(* Logix 5000 AddOnInstructionDefinition export; software revision 16.04 *)

TYPE AKD_Status :   // All connections to the drive ethernet module are established and data is successfully transferring.
STRUCT
   Profile_In_Progress : BOOL;   // Profile Move In Progress
   Block_In_Execution : BOOL;   // Block In Execution
   On_Target_Position : BOOL;   // On Target Position (1=Current Position Equals Last Target Position)
   General_Fault : BOOL;   // General Fault
   Current_Direction : BOOL;   // Current Motor Direction (0=Reverse, 1=Forward)
   Home_Level : BOOL;   // Level of Home Input
   Reg_Level : BOOL;   // Level of Registration Input
   Enable : BOOL;   // State of Enable Output
   Fault_Input_Fault : BOOL;   // Fault Input Active
   Fwd_Limit : BOOL;   // Forward Input Active
   Rev_Limit : BOOL;   // Reverse Input Active
   Positive_Limit : BOOL;   // Positive Software Limit Exceeded
   Negative_Limit : BOOL;   // Negative Software Limit Exceeded
   FE_Fault : BOOL;   // Following Error Fault
   Block_Fault : BOOL;   // Block Execution Fault
   Load_Complete : BOOL;   // Command Message Successfully Loaded
END_STRUCT
END_TYPE

TYPE AKD_Axis :   // Axis Data:
STRUCT
   Control : AKD_Control;   // Control bits to send to the drive
   Status : AKD_Status;   // Status bits received from the drive
   Input : AB:ETHERNET_MODULE_SINT_64Bytes:I:0;   // Data from the drive
   Output : AB:ETHERNET_MODULE_SINT_64Bytes:O:0;   // Data to the drive
   ResponseMsgType : SINT;   // Response type contained in latest IO response from drive. Used to check for errors
   CommandTimeout : INT;   // Time to allow for command response from drive. Dependent on scan rate and communicaiton rate
   PositionFeedback : DINT;   // Actual Position Value
   VelocityFeedback : DINT;   // Actual Velocity Value
END_STRUCT
END_TYPE

TYPE AKD_Control :   // Send Explicit Message
STRUCT
   Load_Data_Start_Profile : BOOL;   // Load Command Data / Start Profile Move
   Start_Block : BOOL;   // Execute Command block or block chain
   Incremental : BOOL;   // Incremental Position (0=Absolute, 1=Incremental)
   Direction : BOOL;   // Direction in Velocity Mode (0=Reverse, 1=Forward)
   Smooth_Stop : BOOL;   // Smooth / Controlled Stop w/ Deceleration
   Hard_Stop : BOOL;   // Hard / Immediate Stop
   Reg_Arm : BOOL;   // Arm the Registration Input
   Enable : BOOL;   // Enable Output
END_STRUCT
END_TYPE

ADD_ON_INSTRUCTION AKD_Set_Attribute   (* revision 2.1, ExecutePrescan, ExecuteEnableInFalse *)
// Set Position Controller Attribute
// Revision note:
// Don't error if Command_Timeout preset is 0
VAR_OUTPUT
   DN : BOOL; {visible}   // Command Successful
   ER : BOOL; {visible}   // Error
END_VAR
VAR_IN_OUT
   Axis : AKD_Axis; {required}
END_VAR
VAR_INPUT
   Attribute_Number : INT; {visible}   // Attribute Number (see help for options)
   Attribute_Value : DINT; {required}   // Attribute Value
END_VAR
VAR
   Command_Timeout : TIMER;   // Timeout Timer
   Command_Message_Type : SINT;   // Command Message Type
   Command_Axis_Number : SINT;   // Command Axis Number
   Step : SINT;
   Command_Bytes : SINT[8];
   OS_LoadStart : BOOL;
END_VAR

ROUTINE EnableInFalse   (* ladder *)
// EnableIn_False
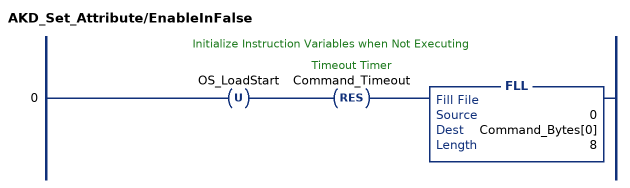
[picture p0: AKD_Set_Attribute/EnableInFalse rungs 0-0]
   // Initialize Instruction Variables when Not Executing
   0: OTU(OS_LoadStart)RES(Command_Timeout)FLL(0,Command_Bytes[0],8);
END_ROUTINE

ROUTINE Logic   (* ladder *)
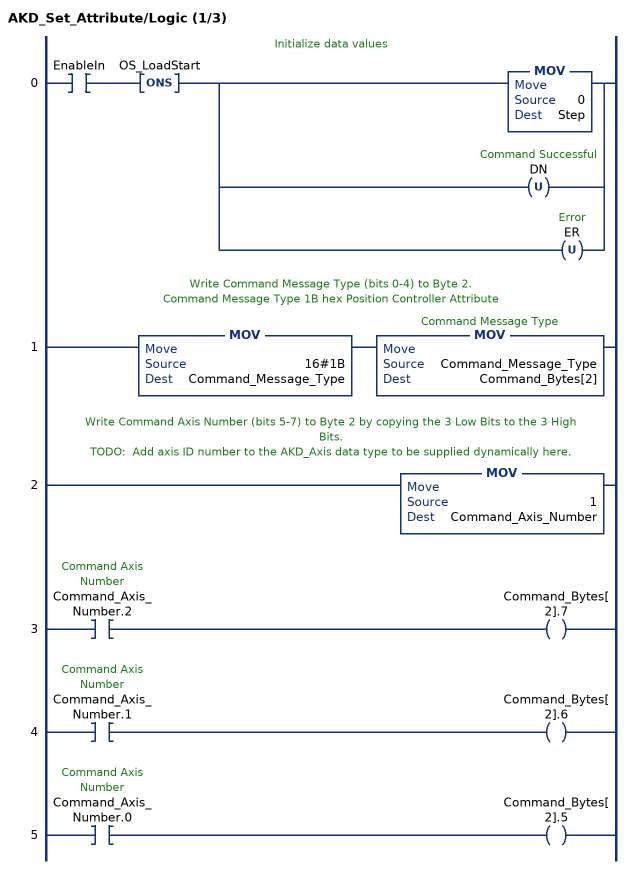
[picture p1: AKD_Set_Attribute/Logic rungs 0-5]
   // Initialize data values
   0: XIC(EnableIn)ONS(OS_LoadStart)[MOV(0,Step) ,OTU(DN) ,OTU(ER) ];
   // Write Command Message Type (bits 0-4) to Byte 2.
   // Command Message Type 1B hex Position Controller Attribute
   1: MOV(16#1B,Command_Message_Type)MOV(Command_Message_Type,Command_Bytes[2]);
   // Write Command Axis Number (bits 5-7) to Byte 2 by copying the 3 Low Bits to the 3 High Bits.
   // TODO:  Add axis ID number to the AKD_Axis data type to be supplied dynamically here.
   2: MOV(1,Command_Axis_Number);
   3: XIC(Command_Axis_Number.2)OTE(Command_Bytes[2].7);
   4: XIC(Command_Axis_Number.1)OTE(Command_Bytes[2].6);
   5: XIC(Command_Axis_Number.0)OTE(Command_Bytes[2].5);
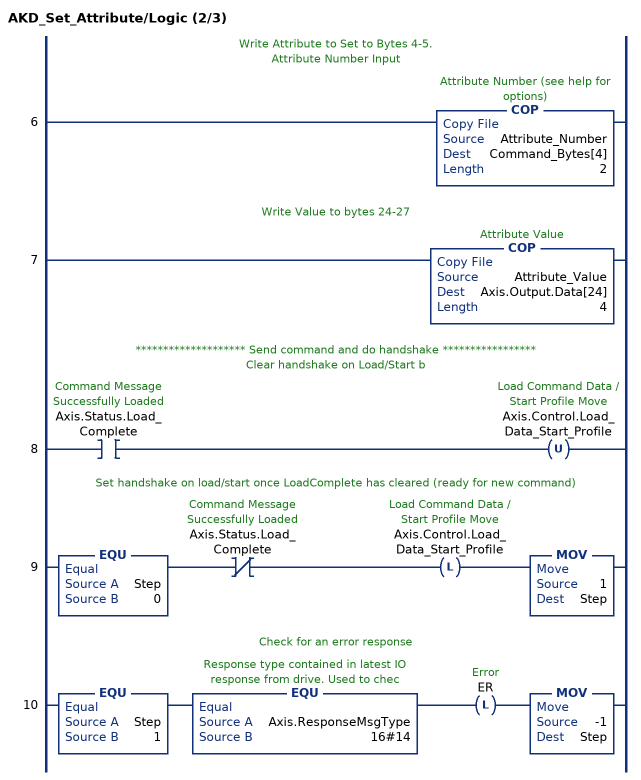
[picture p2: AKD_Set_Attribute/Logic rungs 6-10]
   // Write Attribute to Set to Bytes 4-5.
   // Attribute Number Input
   6: COP(Attribute_Number,Command_Bytes[4],2);
   // Write Value to bytes 24-27
   7: COP(Attribute_Value,Axis.Output.Data[24],4);
   // ******************** Send command and do handshake *****************
   // Clear handshake on Load/Start b
   8: XIC(Axis.Status.Load_Complete)OTU(Axis.Control.Load_Data_Start_Profile);
   // Set handshake on load/start once LoadComplete has cleared (ready for new command)
   9: EQU(Step,0)XIO(Axis.Status.Load_Complete)OTL(Axis.Control.Load_Data_Start_Profile)MOV(1,Step);
   // Check for an error response
   10: EQU(Step,1)EQU(Axis.ResponseMsgType,16#14)OTL(ER)MOV(-1,Step);
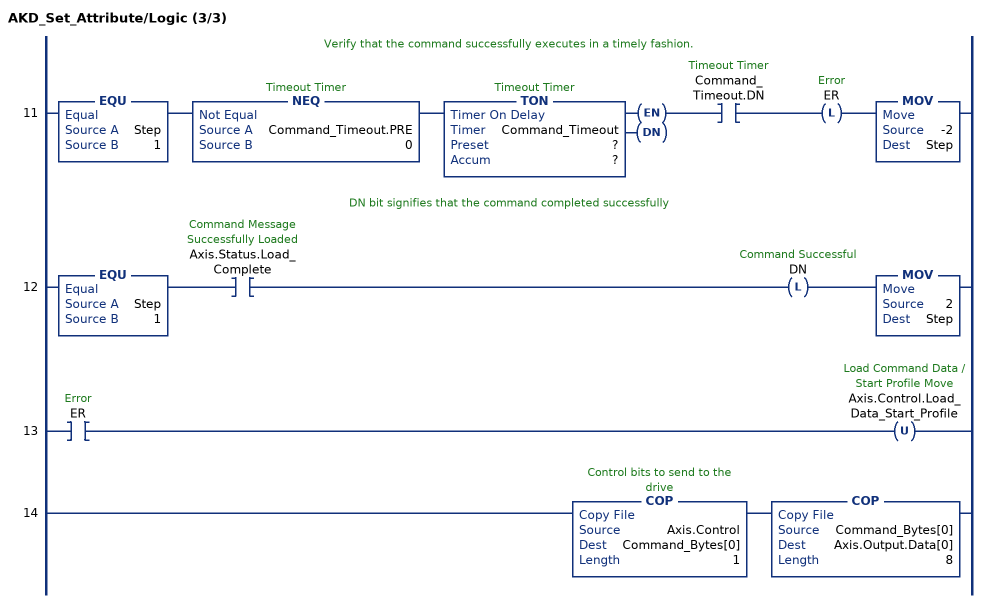
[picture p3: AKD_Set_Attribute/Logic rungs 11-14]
   // Verify that the command successfully executes in a timely fashion.
   11: EQU(Step,1)NEQ(Command_Timeout.PRE,0)TON(Command_Timeout,?,?)XIC(Command_Timeout.DN)OTL(ER)MOV(-2,Step);
   // DN bit signifies that the command completed successfully
   12: EQU(Step,1)XIC(Axis.Status.Load_Complete)OTL(DN)MOV(2,Step);
   13: XIC(ER)OTU(Axis.Control.Load_Data_Start_Profile);
   14: COP(Axis.Control,Command_Bytes[0],1)COP(Command_Bytes[0],Axis.Output.Data[0],8);
END_ROUTINE

ROUTINE Prescan   (* ladder *)
// Prescan
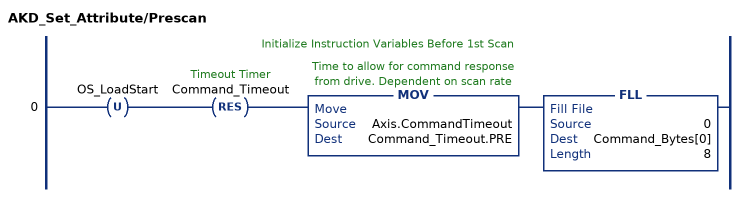
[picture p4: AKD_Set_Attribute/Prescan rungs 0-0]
   // Initialize Instruction Variables Before 1st Scan
   0: OTU(OS_LoadStart)RES(Command_Timeout)MOV(Axis.CommandTimeout,Command_Timeout.PRE)FLL(0,Command_Bytes[0],8);
END_ROUTINE
END_ADD_ON_INSTRUCTION

ADD_ON_INSTRUCTION AKD_Set_Units   (* revision 2.2, ExecutePrescan, ExecuteEnableInFalse *)
// Set Drive Units for Motion Commands
// Revision note:
// Clean up instruction, especially for error recovery.
VAR_IN_OUT
   Axis : AKD_Axis; {required}
END_VAR
VAR_INPUT
   Units : SINT; {required}   // Drive Units (0=Counts 16 bit)
END_VAR
VAR_OUTPUT
   DN : BOOL; {visible}   // Command Successfully Initiated
   ER : BOOL; {visible}   // Error
END_VAR
VAR
   Set_POSUNIT : AKD_Set_Attribute;
   Set_PROFUNIT : AKD_Set_Attribute;
   Step : SINT;   // Sequence Step Number
   OS_Start_Sequence : BOOL;
   Profile_Ratio : DINT;   // The number of actual feedback counts per second or second2 equal to one velocity or acceleration unit
   Position_Ratio : DINT;   // The number of actual position feedback counts equal to one position unit
   Invalid_Input : BOOL;   // Invalid Units Input
END_VAR

ROUTINE EnableInFalse   (* ladder *)
// EnableIn_False
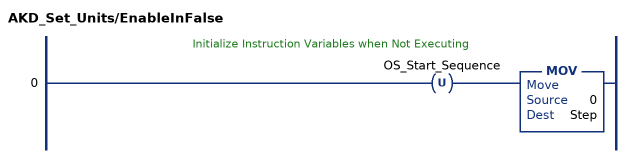
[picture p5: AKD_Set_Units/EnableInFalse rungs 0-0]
   // Initialize Instruction Variables when Not Executing
   0: OTU(OS_Start_Sequence)MOV(0,Step);
END_ROUTINE

ROUTINE Logic   (* ladder *)
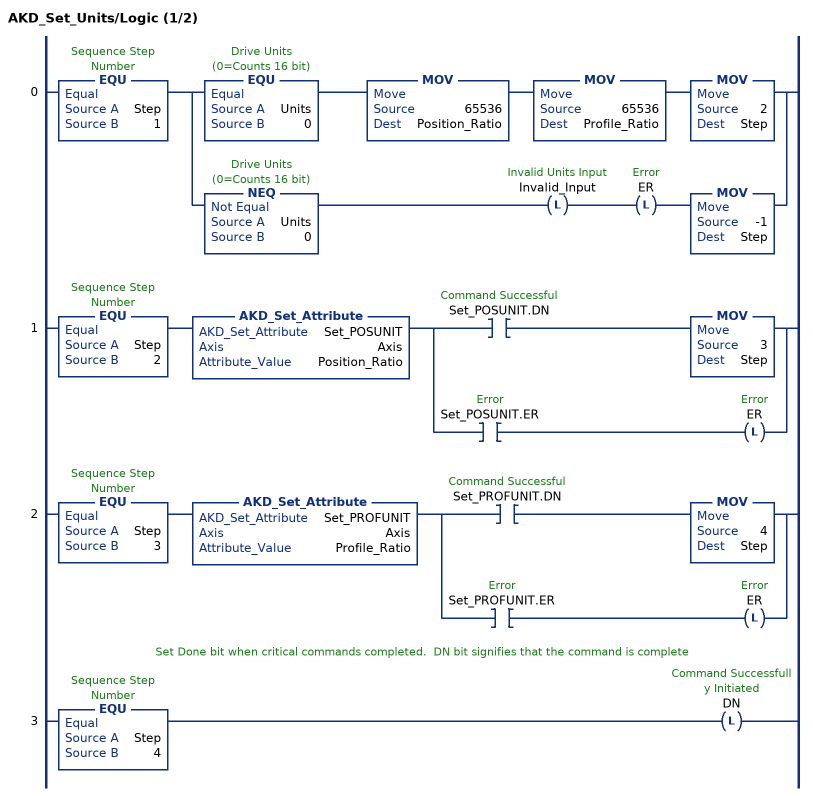
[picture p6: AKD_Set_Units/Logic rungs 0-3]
   0: EQU(Step,1)[EQU(Units,0) MOV(65536,Position_Ratio) MOV(65536,Profile_Ratio) MOV(2,Step) ,NEQ(Units,0) OTL(Invalid_Input) OTL(ER) MOV(-1,Step) ];
   1: EQU(Step,2)AKD_Set_Attribute(Set_POSUNIT,Axis,Position_Ratio)[XIC(Set_POSUNIT.DN) MOV(3,Step) ,XIC(Set_POSUNIT.ER) OTL(ER) ];
   2: EQU(Step,3)AKD_Set_Attribute(Set_PROFUNIT,Axis,Profile_Ratio)[XIC(Set_PROFUNIT.DN) MOV(4,Step) ,XIC(Set_PROFUNIT.ER) OTL(ER) ];
   // Set Done bit when critical commands completed.  DN bit signifies that the command is complete
   3: EQU(Step,4)OTL(DN);
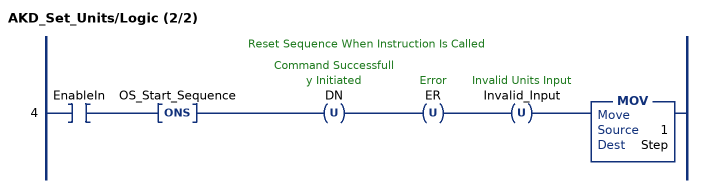
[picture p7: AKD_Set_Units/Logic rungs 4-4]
   // Reset Sequence When Instruction Is Called
   4: XIC(EnableIn)ONS(OS_Start_Sequence)OTU(DN)OTU(ER)OTU(Invalid_Input)MOV(1,Step);
END_ROUTINE

ROUTINE Prescan   (* ladder *)
// Prescan
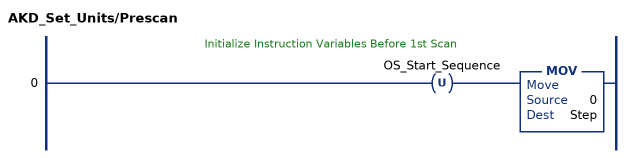
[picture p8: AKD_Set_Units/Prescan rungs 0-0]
   // Initialize Instruction Variables Before 1st Scan
   0: OTU(OS_Start_Sequence)MOV(0,Step);
END_ROUTINE
END_ADD_ON_INSTRUCTION
